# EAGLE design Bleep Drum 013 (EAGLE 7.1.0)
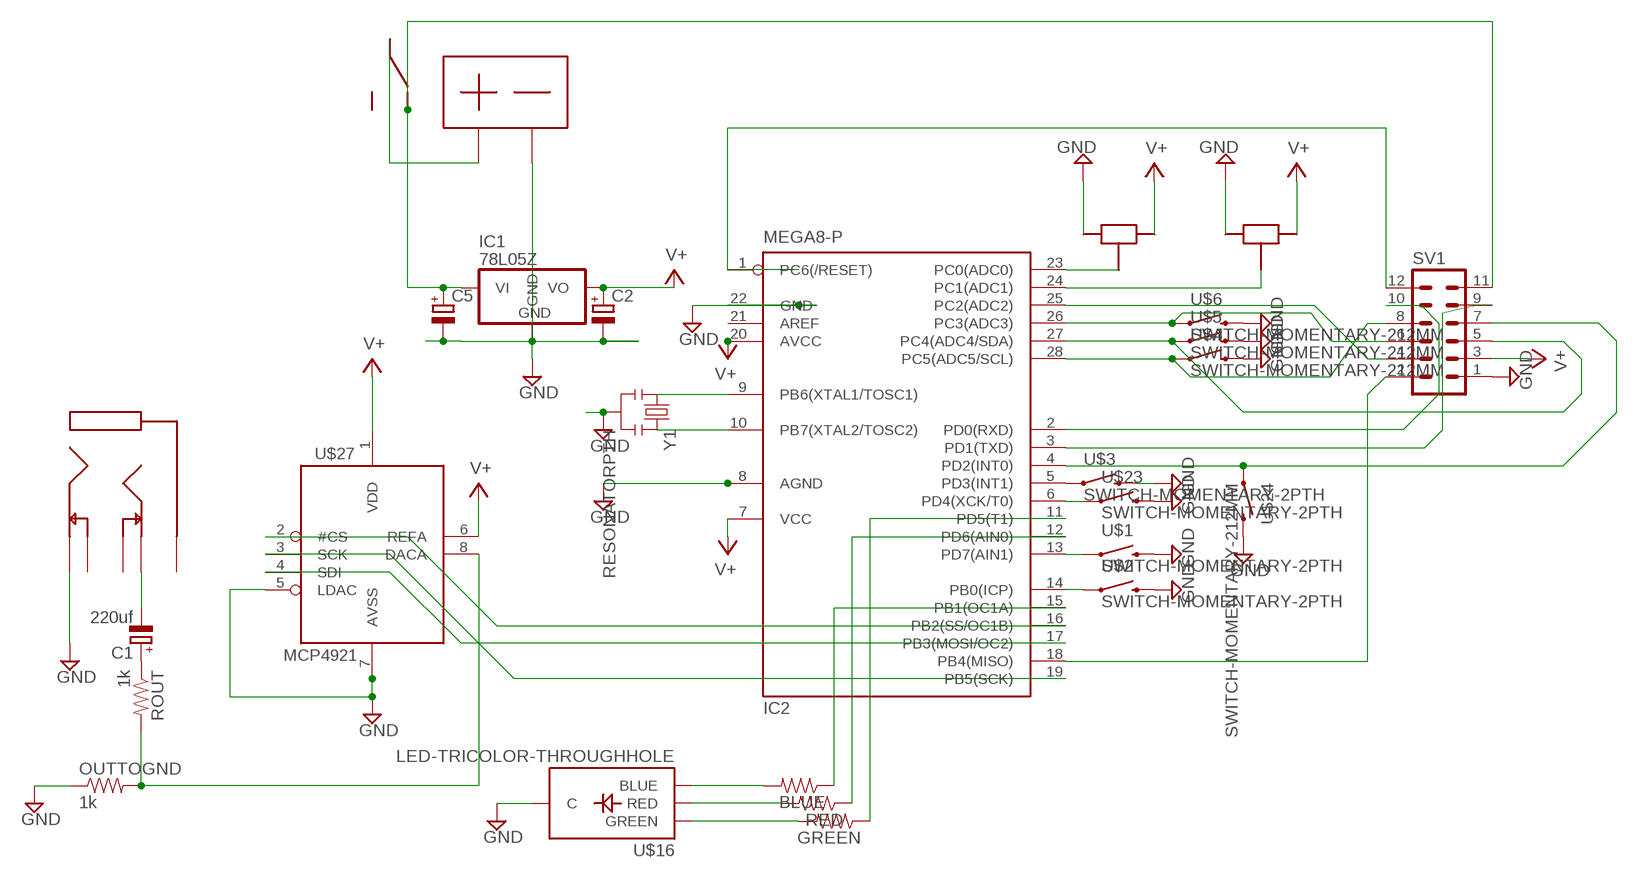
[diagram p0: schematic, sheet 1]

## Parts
BLUE  RESISTORPTH-1/6W  [1/6W-RES]
C1  220uf  CPOL-EUE2.5-6  [E2,5-6]
C2  CPOL-EUE2.5-6  [E2,5-6]
C5  CPOL-EUE2.5-6  [E2,5-6]
GREEN  RESISTORPTH-1/6W  [1/6W-RES]
IC1  78L05Z  [TO92]
IC2  MEGA8-P  [DIL28-3]
OUTTOGND  1k  RESISTORPTH-1/6W  [1/6W-RES]
RED  RESISTORPTH-1/6W  [1/6W-RES]
ROUT  1k  RESISTORPTH-1/6W  [1/6W-RES]
SV1  MA06-2  [MA06-2]
U$1  SWITCH-MOMENTARY-2PTH  [TACTILE-PTH]
U$2  SWITCH-MOMENTARY-2PTH  [TACTILE-PTH]
U$3  SWITCH-MOMENTARY-2PTH  [TACTILE-PTH]
U$4  SWITCH-MOMENTARY-212MM  [TACTILE-PTH-12MM]
U$5  SWITCH-MOMENTARY-212MM  [TACTILE-PTH-12MM]
U$6  SWITCH-MOMENTARY-212MM  [TACTILE-PTH-12MM]
U$7  9VSMALPINS  [9VSMALLPINS]
U$8  1/8STEREO  [1/8STEREO]
U$9  POT  [POT]
U$10  POT  [POT]
U$15  SLIDE_HORIZ_OS  [SLIDE_HORIZ_OS]
U$16  LED-TRICOLOR-THROUGHHOLE  [LED-TRICOLOR-THROUGHHOLE]
U$23  SWITCH-MOMENTARY-2PTH  [TACTILE-PTH]
U$24  SWITCH-MOMENTARY-212MM  [TACTILE-PTH-12MM]
U$27  MCP4921  [DIL08]
Y1  RESONATORPTH  [RESONATOR-PTH]

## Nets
GND: C2.- C5.- IC1.2(GND) IC2.8(AGND) IC2.22(GND) OUTTOGND.1 SV1.1 U$1.3 U$2.3 U$3.3 U$4.3 U$5.3 U$6.3 U$7.P$2 U$8.P$2 U$9.P$3 U$10.P$3 U$16.GND(C) U$23.3 U$24.3 U$27.5(LDAC) U$27.7(AVSS) Y1.2
N$1: IC2.10(PB7(XTAL2/TOSC2)) Y1.3
N$2: BLUE.1 IC2.15(PB1(OC1A))
N$3: IC2.12(PD6(AIN0)) RED.1
N$4: GREEN.1 IC2.11(PD5(T1))
N$5: IC2.1(PC6(/RESET)) SV1.12
N$6: IC2.9(PB6(XTAL1/TOSC1)) Y1.1
N$7: IC2.17(PB3(MOSI/OC2)) U$27.4(SDI)
N$8: U$7.P$1 U$15.P$1
N$9: IC2.19(PB5(SCK)) U$27.3(SCK)
N$10: IC2.23(PC0(ADC0)) U$10.P$2
N$11: IC2.24(PC1(ADC1)) U$9.P$2
N$12: C1.+ ROUT.1
N$13: OUTTOGND.2 ROUT.2 U$27.8(DACA)
N$14: BLUE.2 U$16.GRN(BLUE)
N$15: RED.2 U$16.BLU(RED)
N$16: GREEN.2 U$16.RED(GREEN)
N$17: IC2.5(PD3(INT1)) U$3.1
N$18: C1.- U$8.P$5
N$19: IC2.27(PC4(ADC4/SDA)) SV1.5 U$5.1
N$22: C5.+ IC1.3(VI) SV1.11 U$15.P$2
N$23: C2.+ IC1.1(VO) IC2.7(VCC) IC2.20(AVCC) U$9.P$1 U$10.P$1 U$27.1(VDD) U$27.6(REFA) ; supply symbol labelled V+
N$26: IC2.18(PB4(MISO)) SV1.2
N$28: IC2.14(PB0(ICP)) U$2.1
N$29: IC2.6(PD4(XCK/T0)) U$23.1
N$30: IC2.25(PC2(ADC2)) SV1.4
N$31: IC2.13(PD7(AIN1)) U$1.1
N$32: IC2.2(PD0(RXD)) SV1.10
N$33: IC2.26(PC3(ADC3)) SV1.6 U$6.1
N$34: IC2.28(PC5(ADC5/SCL)) SV1.8 U$4.1
N$35: IC2.3(PD1(TXD)) SV1.9
N$37: IC2.16(PB2(SS/OC1B)) U$27.2(#CS)
P1: IC2.4(PD2(INT0)) SV1.7 U$24.1
V+: SV1.3
Unconnected: IC2.21(AREF) U$8.P$1 U$8.P$3 U$8.P$4 U$15.P$3

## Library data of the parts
BLUE GREEN OUTTOGND RED ROUT = SparkFun-Passives:RESISTOR: Resistor
C1 C2 C5 = rcl:CPOL-EU: POLARIZED CAPACITOR, European symbol
IC1 = linear:78*: Positive VOLTAGE REGULATOR Source: http://cache.national.com/ds/LM/LM78L05.pdf http://www.fairchildsemi.com/ds/LM/LM7805.pdf
IC2 = atmel:MEGA8-P: MICROCONTROLLER 8 Kbytes FLASH, 1 kbytes SRAM, 512 bytes EEPROM, USART, 4-channel 10 bit ADC, 2-channel 8 bit ADC Pin compatible with Atmega48, ATMega88, ATMega168 Source: avr.lbr; OC_FARNELL: unknown; OC_NEWARK: unknown
SV1 = con-lstb:MA06-2: PIN HEADER; OC_FARNELL: unknown; OC_NEWARK: unknown
U$1-U$6 U$23 U$24 = SparkFun-Electromechanical:SWITCH-MOMENTARY-2: Various NO switches- pushbuttons, reed, etc
U$7 = bleep t2:9VSMALPINS
U$8 = bleep t2:1/8STEREO
U$9 U$10 = BLEEP:POT
U$15 = BLEEP:SLIDE_HORIZ_OS
U$16 = SparkFun:LED-TRICOLOR-THROUGHHOLE
U$27 = adafruit:MCP4921
Y1 = SparkFun:RESONATOR: Resonator Small SMD resonator. This is the itty bitty 10/20MHz resonators with built in caps. CSTCE10M0G55 and CSTCE20M0V53. Footprint has been reviewed closely but hasn't been tested yet.

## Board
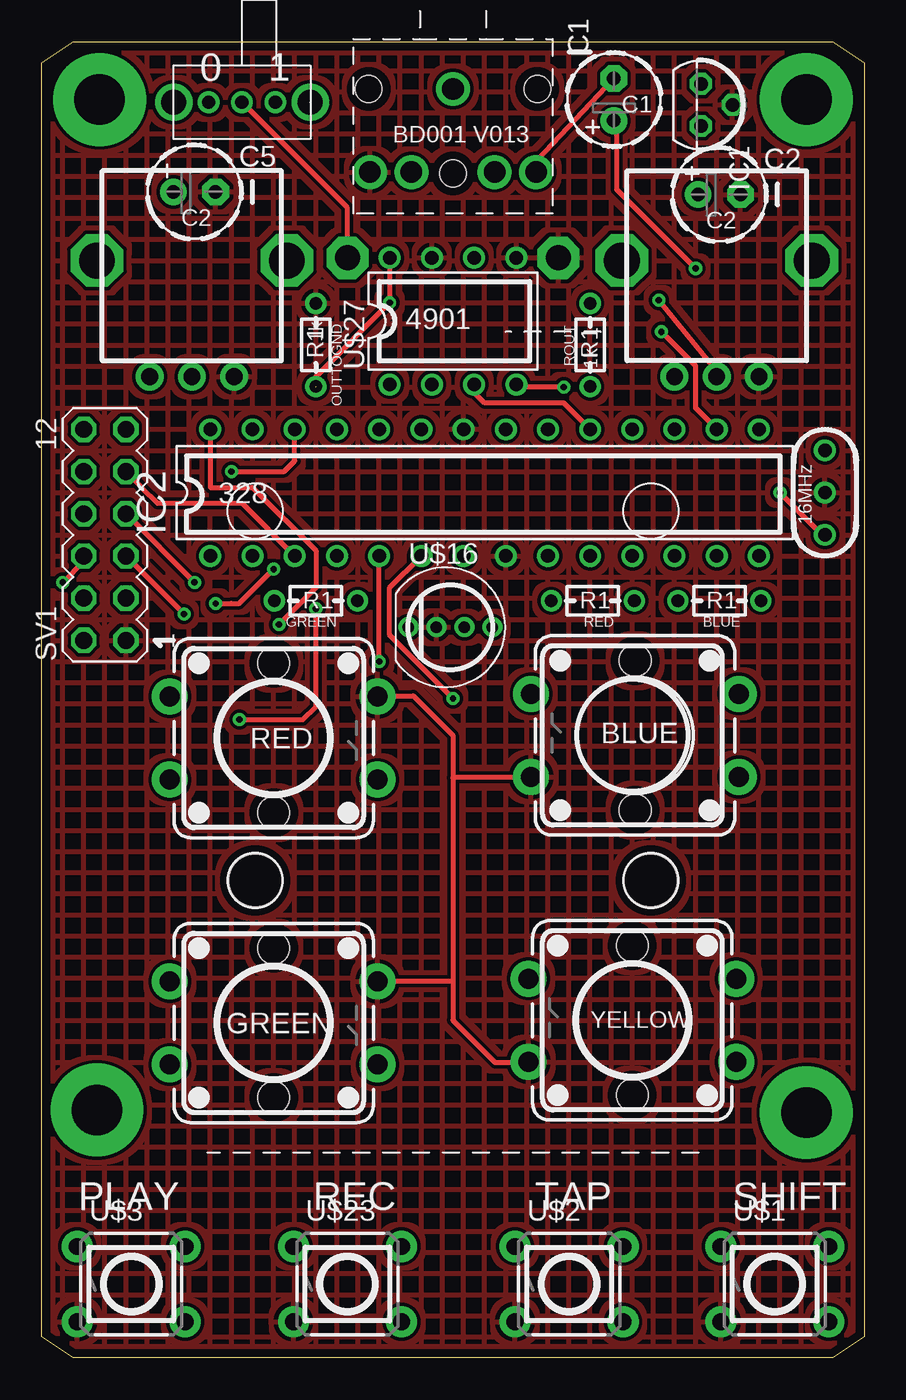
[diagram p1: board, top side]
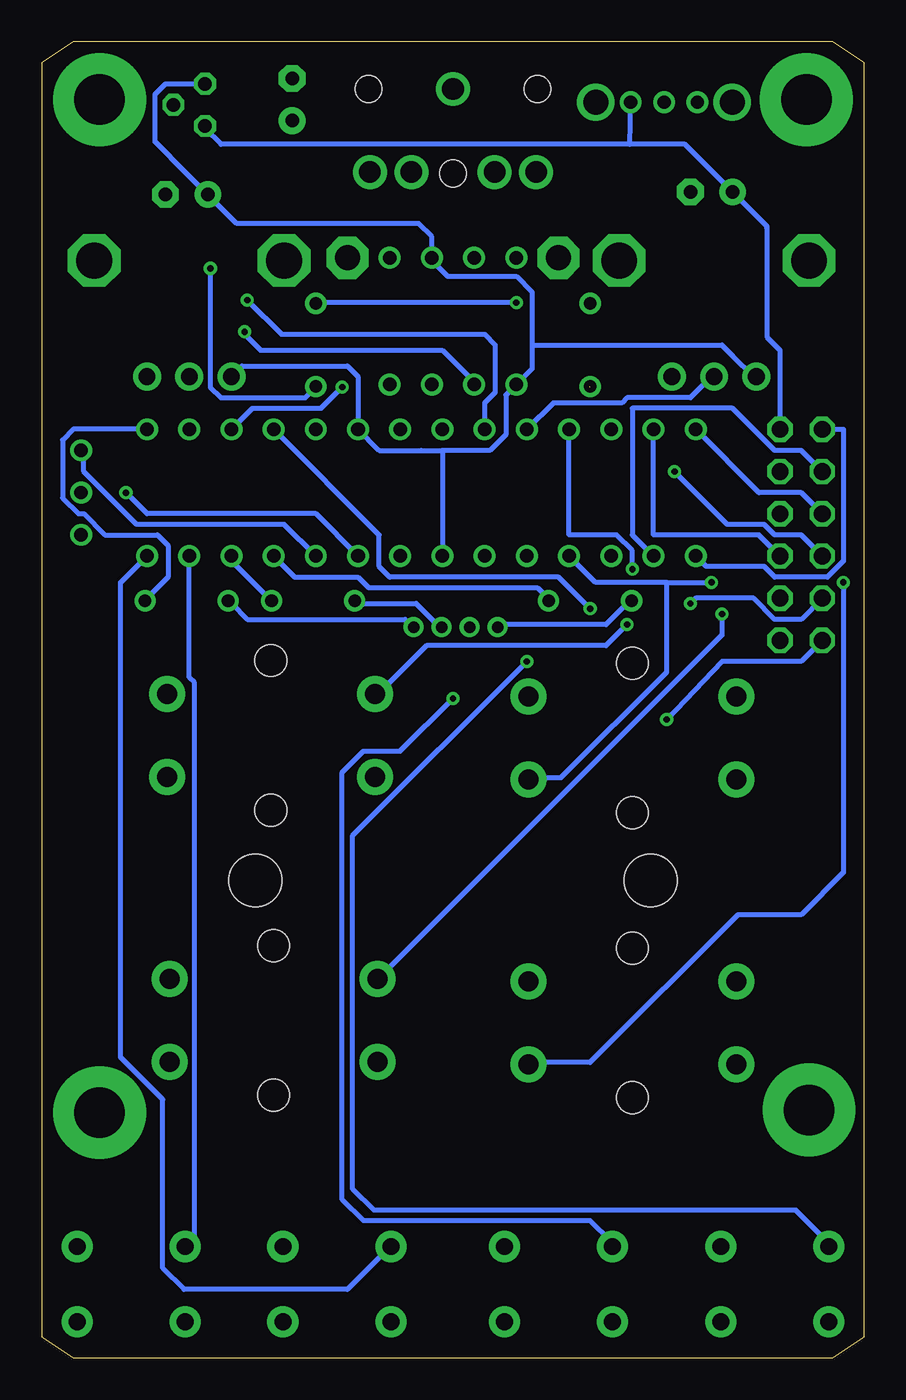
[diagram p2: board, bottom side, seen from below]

Size 49.53 x 79.22 mm. Coordinates in mm from the lower left corner, seen from the top.
Outline: 1.91,79.22 47.62,79.22 49.53,77.95 49.53,1.27 47.62,0 1.91,0 0,1.27 0,77.95 1.91,79.22
Copper layers (1*16): Top 0.035mm / dielectric 1.5mm / Bottom 0.035mm
Design rules "default": minimum track width 12mil, minimum drill 15mil, track to track 8mil, track to pad 8mil, pad to pad 8mil, via to via 8mil, smd to smd 8mil, copper to edge 20mil, drill to drill 8mil, minimum pad ring 10mil, minimum via ring 8mil, stop-mask expansion 4mil, vias tented up to drill 0mil, thermal gap 10mil
Holes 3.17 mm at 12.86,28.73 36.67,28.73

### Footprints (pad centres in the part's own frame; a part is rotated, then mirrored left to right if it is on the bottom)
1/6W-RES = drill 0.762: 1 -2.5,0; 2 2.5,0
E2,5-6 = drill 0.813 pad 1.6: + -1.27,0 | drill 0.813 pad 1.6 octagon: - 1.27,0
TO92 = drill 0.813 octagon: 1 -1.27,0; 2 0,1.905; 3 1.27,0
DIL28-3 = drill 0.813: 1 -16.51,-3.81; 2 -13.97,-3.81; 3 -11.43,-3.81; 4 -8.89,-3.81; 5 -6.35,-3.81; 6 -3.81,-3.81; 7 -1.27,-3.81; 8 1.27,-3.81; 9 3.81,-3.81; 10 6.35,-3.81; 11 8.89,-3.81; 12 11.43,-3.81; 13 13.97,-3.81; 14 16.51,-3.81; 15 16.51,3.81; 16 13.97,3.81; 17 11.43,3.81; 18 8.89,3.81; 19 6.35,3.81; 20 3.81,3.81; 21 1.27,3.81; 22 -1.27,3.81; 23 -3.81,3.81; 24 -6.35,3.81; 25 -8.89,3.81; 26 -11.43,3.81; 27 -13.97,3.81; 28 -16.51,3.81
MA06-2 = drill 1.016 octagon: 1 -6.35,-1.27; 2 -6.35,1.27; 3 -3.81,-1.27; 4 -3.81,1.27; 5 -1.27,-1.27; 6 -1.27,1.27; 7 1.27,-1.27; 8 1.27,1.27; 9 3.81,-1.27; 10 3.81,1.27; 11 6.35,-1.27; 12 6.35,1.27
TACTILE-PTH = drill 1.016 pad 1.88: 1 -3.251,2.261; 2 3.251,2.261; 3 -3.251,-2.261; 4 3.251,-2.261
TACTILE-PTH-12MM = drill 1.2 pad 2.159: 1 6.25,-2.5; 2 -6.25,-2.5; 3 6.25,2.5; 4 -6.25,2.5 | hole 1.905: 0,4.5; 0,-4.5
9VSMALLPINS = drill 1.5 pad 2.54 octagon: P$1 0,-6.35; P$2 0,6.35
1/8STEREO = drill 1.3 pad 2.032: P$1 0,0; P$2 5,-5; P$3 5,-2.5; P$4 5,2.5; P$5 5,5 | hole 1.6: 0,5.08; 5.08,0; 0,-5.08
POT = drill 1 pad 1.676: P$1 -2.54,-6.985; P$2 0,-6.985; P$3 2.54,-6.985 | drill 2.159 octagon: P$7 -5.715,0; P$8 5.715,0
SLIDE_HORIZ_OS = drill 0.8: P$1 0,0; P$2 2.007,0; P$3 -2.007,0 | drill 1.5 pad 2.032: P$4 4.102,0; P$5 -4.102,0
LED-TRICOLOR-THROUGHHOLE = drill 0.7: BLU 0.841,0; GND -0.841,0; GRN 2.524,0; RED -2.524,0
DIL08 = drill 0.813: 1 -3.81,-3.81; 2 -1.27,-3.81; 3 1.27,-3.81; 4 3.81,-3.81; 5 3.81,3.81; 6 1.27,3.81; 7 -1.27,3.81; 8 -3.81,3.81
RESONATOR-PTH = drill 0.8 pad 1.27: 1 -2.54,0; 2 0,0; 3 2.54,0

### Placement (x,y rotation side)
BLUE  40.8,45.56 180 top
C1  34.45,75.72 90 top
C2  40.8,70.01 0 top
C5  9.21,70.17 0 top
GREEN  16.51,45.56 180 top
IC1  39.69,75.41 270 top
IC2  26.67,52.07 0 top
OUTTOGND  16.51,60.96 270 top
RED  33.18,45.56 180 top
ROUT  33.02,60.96 90 top
SV1  3.81,49.53 90 top
U$1  44.13,4.45 0 top
U$2  31.75,4.45 0 top
U$3  5.4,4.45 0 top
U$4  35.72,37.47 180 top
U$5  35.56,20.32 180 top
U$6  13.97,20.16 0 top
U$7  24.77,66.2 270 top
U$8  24.77,76.36 270 top
U$9  9.05,66.04 0 top
U$10  40.64,66.04 0 top
U$15  12.06,75.56 0 top
U$16  24.61,43.97 0 top
U$23  18.41,4.45 0 top
U$24  13.97,37.31 0 top
U$27  24.77,62.39 0 top
Y1  47.15,52.07 90 top

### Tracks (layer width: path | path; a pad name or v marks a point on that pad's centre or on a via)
GND
  pour Top (hatched): 0,0 0,79.22 49.53,79.22 49.53,0
N$1
  Bottom 0.305: IC2.10 34.92,50.16 43.81,50.16 46.99,53.34 46.99,54.61 Y1.3
N$2
  Bottom 0.305: IC2.15 47.62,55.88 48.26,55.24 48.26,51.75 47.31,50.8 46.99,50.8 45.72,49.53 42.55,49.53 41.91,48.9 41.91,46.99 43.18,45.72 BLUE.1
N$3
  Bottom 0.305: IC2.12 38.1,47.94 35.88,45.72 RED.1
N$4
  Bottom 0.305: IC2.11 34.29,46.99 30.48,46.99 29.84,46.35 19.68,46.35 19.05,45.72 GREEN.1
N$5
  Bottom 0.305: IC2.1 9.53,47.62 6.03,47.62 5.4,46.99 2.22,46.99 1.27,47.94 1.27,55.88 SV1.12
N$6  (via drill 0.38)
  Top 0.305: v44.45,52.07 46.99,49.53 Y1.1
  Bottom 0.305: v44.45,52.07 43.18,50.8 33.02,50.8 IC2.9
N$7  (via drill 0.38)
  Top 0.305: v31.43,58.42 28.57,58.42 U$27.4
  Bottom 0.305: v31.43,58.42 32.7,57.15 36.83,57.15 IC2.17
N$8
  Top 0.305: U$15.P$1 18.41,69.22 18.41,66.36 U$7.P$1
N$9
  Top 0.305: U$27.3 26.04,58.1 26.67,57.47 31.43,57.47 IC2.19
N$10  (via drill 0.38)
  Top 0.305: v37.15,63.66 40.64,59.37 U$10.P$2
  Bottom 0.305: IC2.23 22.86,57.47 22.23,58.1 22.23,60.96 22.86,61.59 35.08,61.59 v37.15,63.66
N$11
  Bottom 0.305: U$9.P$2 9.21,59.05 10.48,57.78 14.29,57.78 14.61,57.47 18.73,57.47 IC2.24
N$12  (via drill 0.38)
  Top 0.305: v39.37,65.56 34.61,70.33 34.61,73.98 C1.+
  Bottom 0.305: v39.37,65.56 39.37,63.18 39.37,58.42 38.73,57.78 33.66,57.78 33.02,58.42 ROUT.1
N$13  (via drill 0.38)  (1 unrouted)
  Top 0.305: 20.95,66.04 U$27.8 20.95,66.04 | 16.51,58.42 16.51,59.05 v20.95,63.5 20.95,66.04
  Bottom 0.305: v20.95,63.5 33.02,63.5 ROUT.2
N$14
  Bottom 0.305: U$16.GRN 27.3,44.13 27.62,44.45 37.15,44.45 38.1,45.4 BLUE.2
N$15
  Bottom 0.305: U$16.BLU 25.72,44.13 26.99,45.4 30.48,45.4 RED.2
N$16
  Bottom 0.305: U$16.RED 21.91,44.13 15.56,44.13 14.29,45.4 GREEN.2
N$17  (via drill 0.38)
  Top 0.305: v20.32,41.91 IC2.5
  Bottom 0.305: v20.32,41.91 30.8,31.43 30.8,10.16 29.53,8.89 4.13,8.89 2.22,6.99 U$3.1
N$18
  Top 0.305: C1.- 29.84,72.07 U$8.P$5
N$19  (via drill 0.38)
  Top 0.305: SV1.5 v8.57,44.77
  Bottom 0.305: IC2.27 12.7,49.53 6.35,49.53 SV1.5 | v8.57,44.77 8.57,43.5 10.79,41.27 12.7,39.37 29.21,22.86 U$5.1
N$20
  Top 0.305: 20.16,39.85 22.38,39.85 24.77,37.47 24.77,34.92 | 24.77,34.92 24.77,22.7 | 24.77,22.7 24.77,20.32 27.3,17.78 29.37,17.78 | 20.32,22.7 24.77,22.7 | 29.53,34.92 24.77,34.92
N$21  (via drill 3.05 pad 5.59)
  other vias: 46.04,75.72
N$22
  Bottom 0.305: 10.79,73.03 8.41,70.64 C5.+ 5.87,68.1 | 10.79,73.03 14.13,73.03 | 14.13,73.03 U$15.P$2 | 10.79,73.03 14.13,73.03 | 14.13,73.03 38.73,73.03 39.69,73.98 IC1.3 | SV1.11 5.08,60.64 5.87,61.44 5.87,67.94 | 5.87,68.1 5.87,67.94 | 5.87,67.94 5.87,68.1 | 5.87,68.1 5.87,67.94
N$23
  Bottom 0.305: 25.4,54.61 IC2.7 | 25.4,54.61 26.67,54.61 29.21,54.61 IC2.20 30.48,59.05 31.11,59.69 37.47,59.69 U$10.P$1 | 40.8,71.28 42.7,73.18 42.7,76.04 42.07,76.68 39.53,76.68 IC1.1 | 40.8,71.28 C2.+ 40.8,71.28 | 26.04,66.04 25.08,65.09 20.95,65.09 20,64.14 20,60.96 | U$9.P$1 6.67,59.05 7.94,60.33 8.57,60.96 20,60.96 | 40.8,71.28 37.78,68.26 26.83,68.26 26.04,67.47 26.04,66.04 | 26.04,66.04 U$27.6 | 20,60.96 20,59.53 U$27.1 21.59,57.94 21.59,55.56 22.54,54.61 25.4,54.61
N$24  (via drill 3.05 pad 5.59)
  other vias: 46.04,14.76
N$25  (via drill 3.05 pad 5.59)
  other vias: 3.33,14.92
N$26  (via drill 0.38)
  Top 0.305: v11.91,38.42 15.72,38.42 16.51,39.21 v16.51,45.09
  Bottom 0.305: v16.51,45.09 18.41,46.99 28.57,46.99 29.21,47.62 29.21,49.53 IC2.18 | v11.91,38.42 8.57,41.91 3.81,41.91 SV1.2
N$28
  Bottom 0.305: IC2.14 44.77,46.67 44.77,18.1 42.23,15.56 42.23,5.4 40.96,4.13 31.11,4.13 28.57,6.67 U$2.1
N$29  (via drill 0.38)
  Top 0.305: IC2.6 20.95,46.35 20.95,43.5 v24.77,39.69
  Bottom 0.305: v24.77,39.69 27.94,36.51 30.16,36.51 31.43,35.24 31.43,9.53 30.16,8.26 16.51,8.26 15.24,6.99 U$23.1
N$30  (via drill 0.38)
  Top 0.305: v10.48,45.4 11.43,45.4 11.91,45.4 v13.97,47.47
  Bottom 0.305: IC2.25 17.78,49.53 14.92,49.53 13.97,48.58 v13.97,47.47 | v10.48,45.4 10.16,45.72 6.67,45.72 5.4,44.45 3.81,44.45 SV1.4
N$31
  Bottom 0.305: IC2.13 40.64,40.96 40.32,40.64 40.32,6.99 40.64,6.99 U$1.1
N$32
  Bottom 0.305: IC2.2 13.97,49.53 13.97,57.15 7.94,57.15 5.4,54.61 3.81,54.61 SV1.10
N$33  (via drill 0.38)
  Top 0.305: v11.43,53.34 14.61,53.34 15.24,53.98 IC2.26 | v1.27,46.67 2.54,47.94 SV1.6
  Bottom 0.305: v11.43,53.34 8.26,50.16 6.03,50.16 5.4,49.53 3.81,49.53 SV1.6 | v1.27,46.67 1.27,36.51 1.27,29.21 3.81,26.67 7.62,26.67 16.51,17.78 20,17.78 U$6.1
N$34  (via drill 0.38)
  Top 0.305: v14.29,44.13 16.51,46.35 16.51,48.58 12.7,52.39 10.16,52.39 IC2.28
  Bottom 0.305: IC2.28 6.35,52.07 3.81,52.07 SV1.8 | v14.29,44.13 15.56,42.86 26.35,42.86 29.21,40.01 U$4.1
N$35
  Top 0.305: IC2.3 12.06,51.44 6.99,51.44 6.03,52.39 SV1.9
N$37  (via drill 0.38)
  Top 0.305: v37.31,61.75 38.42,60.64 39.37,59.69 39.37,57.15 IC2.16
  Bottom 0.305: v37.31,61.75 37.31,61.59 36.35,60.64 25.4,60.64 23.5,58.74 U$27.2
N$89  (via drill 3.05 pad 5.59)
  other vias: 3.49,75.72
P1  (via drill 0.38)
  Top 0.305: v9.21,46.67 SV1.7
  Bottom 0.305: IC2.4 16.19,46.67 11.91,46.67 | 11.91,46.67 11.91,44.29 11.91,41.27 18.26,34.92 20,34.92 U$24.1 | v9.21,46.67 9.53,46.67 11.91,46.67

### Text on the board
_tsilk: 0 | 1 | C1 | BD001 V013 | C2 | C2 | 4901 | R1 | R1 | 328 | 16MHz | R1 | R1 | R1 | RED | BLUE | GREEN | YELLOW | PLAY | REC | TAP | SHIFT

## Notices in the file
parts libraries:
SparkFun-Passives: Licensing: CC v3.0 Share-Alike You are welcome to use this library for commercial purposes.
